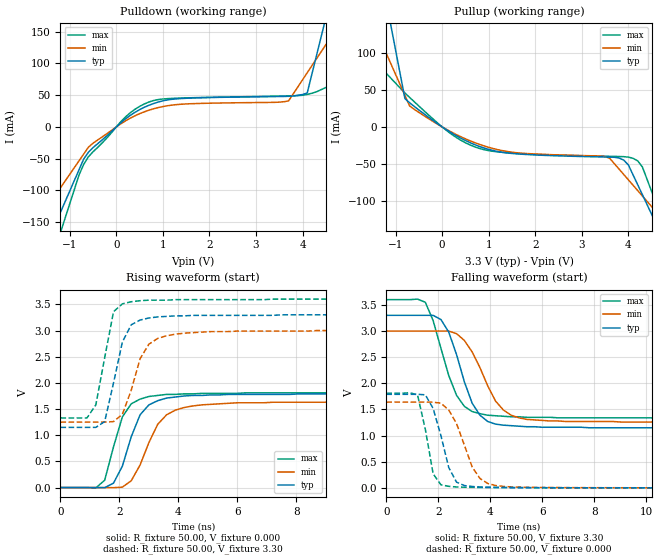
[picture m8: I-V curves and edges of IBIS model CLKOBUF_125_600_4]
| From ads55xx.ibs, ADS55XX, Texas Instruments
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|   Model CLKOBUF_125_600_4
[Model]   CLKOBUF_125_600_4
Model_type   Output
Polarity   Non-Inverting
Vmeas =   1.65V
C_comp   2pf   2pf   2pf
[Temperature Range]   50.00   0.10k   -20.00
[Voltage Range]   3.30V   3.00V   3.60V
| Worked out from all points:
|   slope of the pulldown table from 0 to 0.495 V, typ, clamps not added: 18.3 ohm
|   slope of the pullup table from 0 to 0.495 V, typ, clamps not added: 27.2 ohm
|   rising waveform, R_fixture 50.00, V_fixture 0.000: 20-80 % time 714ps typ, 872ps min, 614ps max; typ from 0 V to 1.79 V
|   rising waveform, R_fixture 50.00, V_fixture 3.30: 20-80 % time 552ps typ, 673ps min, 459ps max; typ from 1.15 V to 3.3 V
|   falling waveform, R_fixture 50.00, V_fixture 3.30: 20-80 % time 875ps typ, 1.06ns min, 858ps max; typ from 3.3 V to 1.15 V
|   falling waveform, R_fixture 50.00, V_fixture 0.000: 20-80 % time 583ps typ, 792ps min, 416ps max; typ from 1.79 V to 0.001 V
[Pulldown]
| voltage   I(typ)   I(min)   I(max)
-3.3V     -487.8mA   -319.5mA   -643.9mA
-1.9V     -252.3mA   -170.4mA   -325.6mA
-1.5V     -185mA     -127.8mA   -234.6mA
-1V       -100.9mA   -74.57mA   -120.9mA
-600mV    -39.98mA   -31.97mA   -47.03mA
700mV     34.09mA    26.33mA    39.24mA
3.7V      48.24mA    41.07mA    48.88mA
4V        51.08mA    74.25mA    49.9mA
4.1V      53.43mA    85.31mA    51.16mA
4.5V      171.9mA    129.6mA    62.06mA
4.9V      290.3mA    173.8mA    75.4mA
6.6V      793.7mA    361.8mA    132.1mA
[Pullup]
| voltage   I(typ)   I(min)   I(max)
-3.3V     855.5mA    396.5mA    211.5mA
-2.1V     463.2mA    226.6mA    131.9mA
-1.5V     267.1mA    141.7mA    92.17mA
-1V       103.6mA    70.86mA    59.02mA
-800mV    38.24mA    42.54mA    45.76mA
-700mV    32.59mA    28.38mA    39.89mA
600mV     -21.26mA   -18.74mA   -24.36mA
3.5V      -40.58mA   -40.01mA   -39.53mA
4.1V      -64.7mA    -78.67mA   -42.39mA
4.5V      -118.1mA   -107.6mA   -87.19mA
4.9V      -171.5mA   -136.6mA   -153.6mA
6.6V      -398.4mA   -259.7mA   -436mA
[Ramp]
| variable   typ   min   max
dV/dt_r   1.07/0.68n   0.98/0.82n   1.09/0.57n
dV/dt_f   1.29/0.85n   1.05/1.03n   1.36/0.85n
R_load = 50.00
[Rising Waveform]
R_fixture = 50.00
V_fixture = 0.000
V_fixture_min = 0.000
V_fixture_max = 0.000
| time   V(typ)   V(min)   V(max)
0s        24.28nV    34.14nV    47.47nV
1.2ns     -9.99uV    590nV      -5.74mV
1.5ns     -2.78mV    36.32uV    140mV
1.8ns     84.95mV    -2.25mV    780mV
2.1ns     410mV      8.38mV     1.35V
2.4ns     970mV      130mV      1.6V
3ns       1.58V      860mV      1.74V
3.6ns     1.71V      1.39V      1.78V
4.8ns     1.76V      1.58V      1.8V
15ns      1.79V      1.64V      1.81V
[Rising Waveform]
R_fixture = 50.00
V_fixture = 3.30
V_fixture_min = 3.00
V_fixture_max = 3.60
| time   V(typ)   V(min)   V(max)
0s        1.15V      1.25V      1.33V
900ps     1.15V      1.25V      1.33V
1.2ns     1.15V      1.25V      1.58V
1.5ns     1.26V      1.25V      2.48V
1.8ns     2V         1.26V      3.36V
2.1ns     2.78V      1.4V       3.51V
2.7ns     3.2V       2.46V      3.57V
3ns       3.24V      2.74V      3.58V
3.6ns     3.27V      2.9V       3.58V
15ns      3.3V       3V         3.6V
[Falling Waveform]
R_fixture = 50.00
V_fixture = 3.30
V_fixture_min = 3.00
V_fixture_max = 3.60
| time   V(typ)   V(min)   V(max)
0s        3.3V       3V         3.6V
1.5ns     3.3V       3V         3.55V
2.1ns     3.22V      3V         2.67V
2.4ns     2.98V      3V         2.15V
2.7ns     2.55V      2.95V      1.77V
3.3ns     1.62V      2.6V       1.46V
3.6ns     1.39V      2.3V       1.42V
4.2ns     1.22V      1.66V      1.38V
5.1ns     1.18V      1.34V      1.36V
15ns      1.15V      1.26V      1.33V
[Falling Waveform]
R_fixture = 50.00
V_fixture = 0.000
V_fixture_min = 0.000
V_fixture_max = 0.000
| time   V(typ)   V(min)   V(max)
0s        1.79V      1.64V      1.81V
1.2ns     1.79V      1.64V      1.78V
1.5ns     1.78V      1.64V      1.12V
1.8ns     1.52V      1.64V      270mV
2.1ns     1V         1.62V      59.82mV
2.4ns     390mV      1.49V      29.68mV
2.7ns     110mV      1.23V      18.37mV
3.3ns     26.86mV    400mV      9.89mV
4.2ns     10.66mV    45.8mV     5.83mV
15ns      940uV      1.3mV      950uV
